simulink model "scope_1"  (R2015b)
settings: Solver=ode45  StartTime=0.0  StopTime=10.0  RelTol=1e-3
undefined symbols (not defined in the file or in its folder): fir1

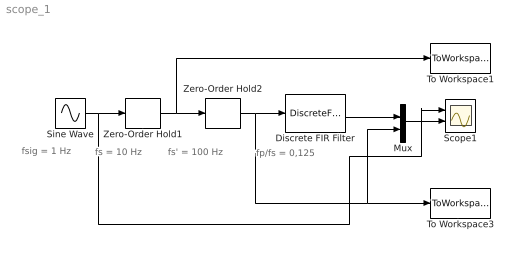
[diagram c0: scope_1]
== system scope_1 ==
  note: fsig = 1 Hz
  note: fp/fs = 0,125
  note: fs' = 100 Hz
  note: fs = 10 Hz
  Discrete FIR Filter : DiscreteFir  Coefficients=fir1(128,0.025)
  Mux : Mux  Inputs=2
  Scope1 : Scope  NumInputPorts=2
  Sine Wave : Sin  Frequency=2*pi*1  SampleTime=0
  To Workspace1 : ToWorkspace  VariableName=y2  SaveFormat=Timeseries  SampleTime=-1
  To Workspace3 : ToWorkspace  VariableName=y1  SaveFormat=Timeseries  SampleTime=-1
  Zero-Order Hold1 : ZeroOrderHold  SampleTime=0.1
  Zero-Order Hold2 : ZeroOrderHold  SampleTime=1/100
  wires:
  Mux/1 -> Scope1/2
  Sine Wave/1 -> Scope1/1, Zero-Order Hold1/1
  Zero-Order Hold2/1 -> Mux/2, To Workspace3/1, Discrete FIR Filter/1
  Zero-Order Hold1/1 -> To Workspace1/1, Zero-Order Hold2/1
  Discrete FIR Filter/1 -> Mux/1
